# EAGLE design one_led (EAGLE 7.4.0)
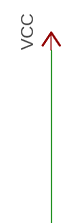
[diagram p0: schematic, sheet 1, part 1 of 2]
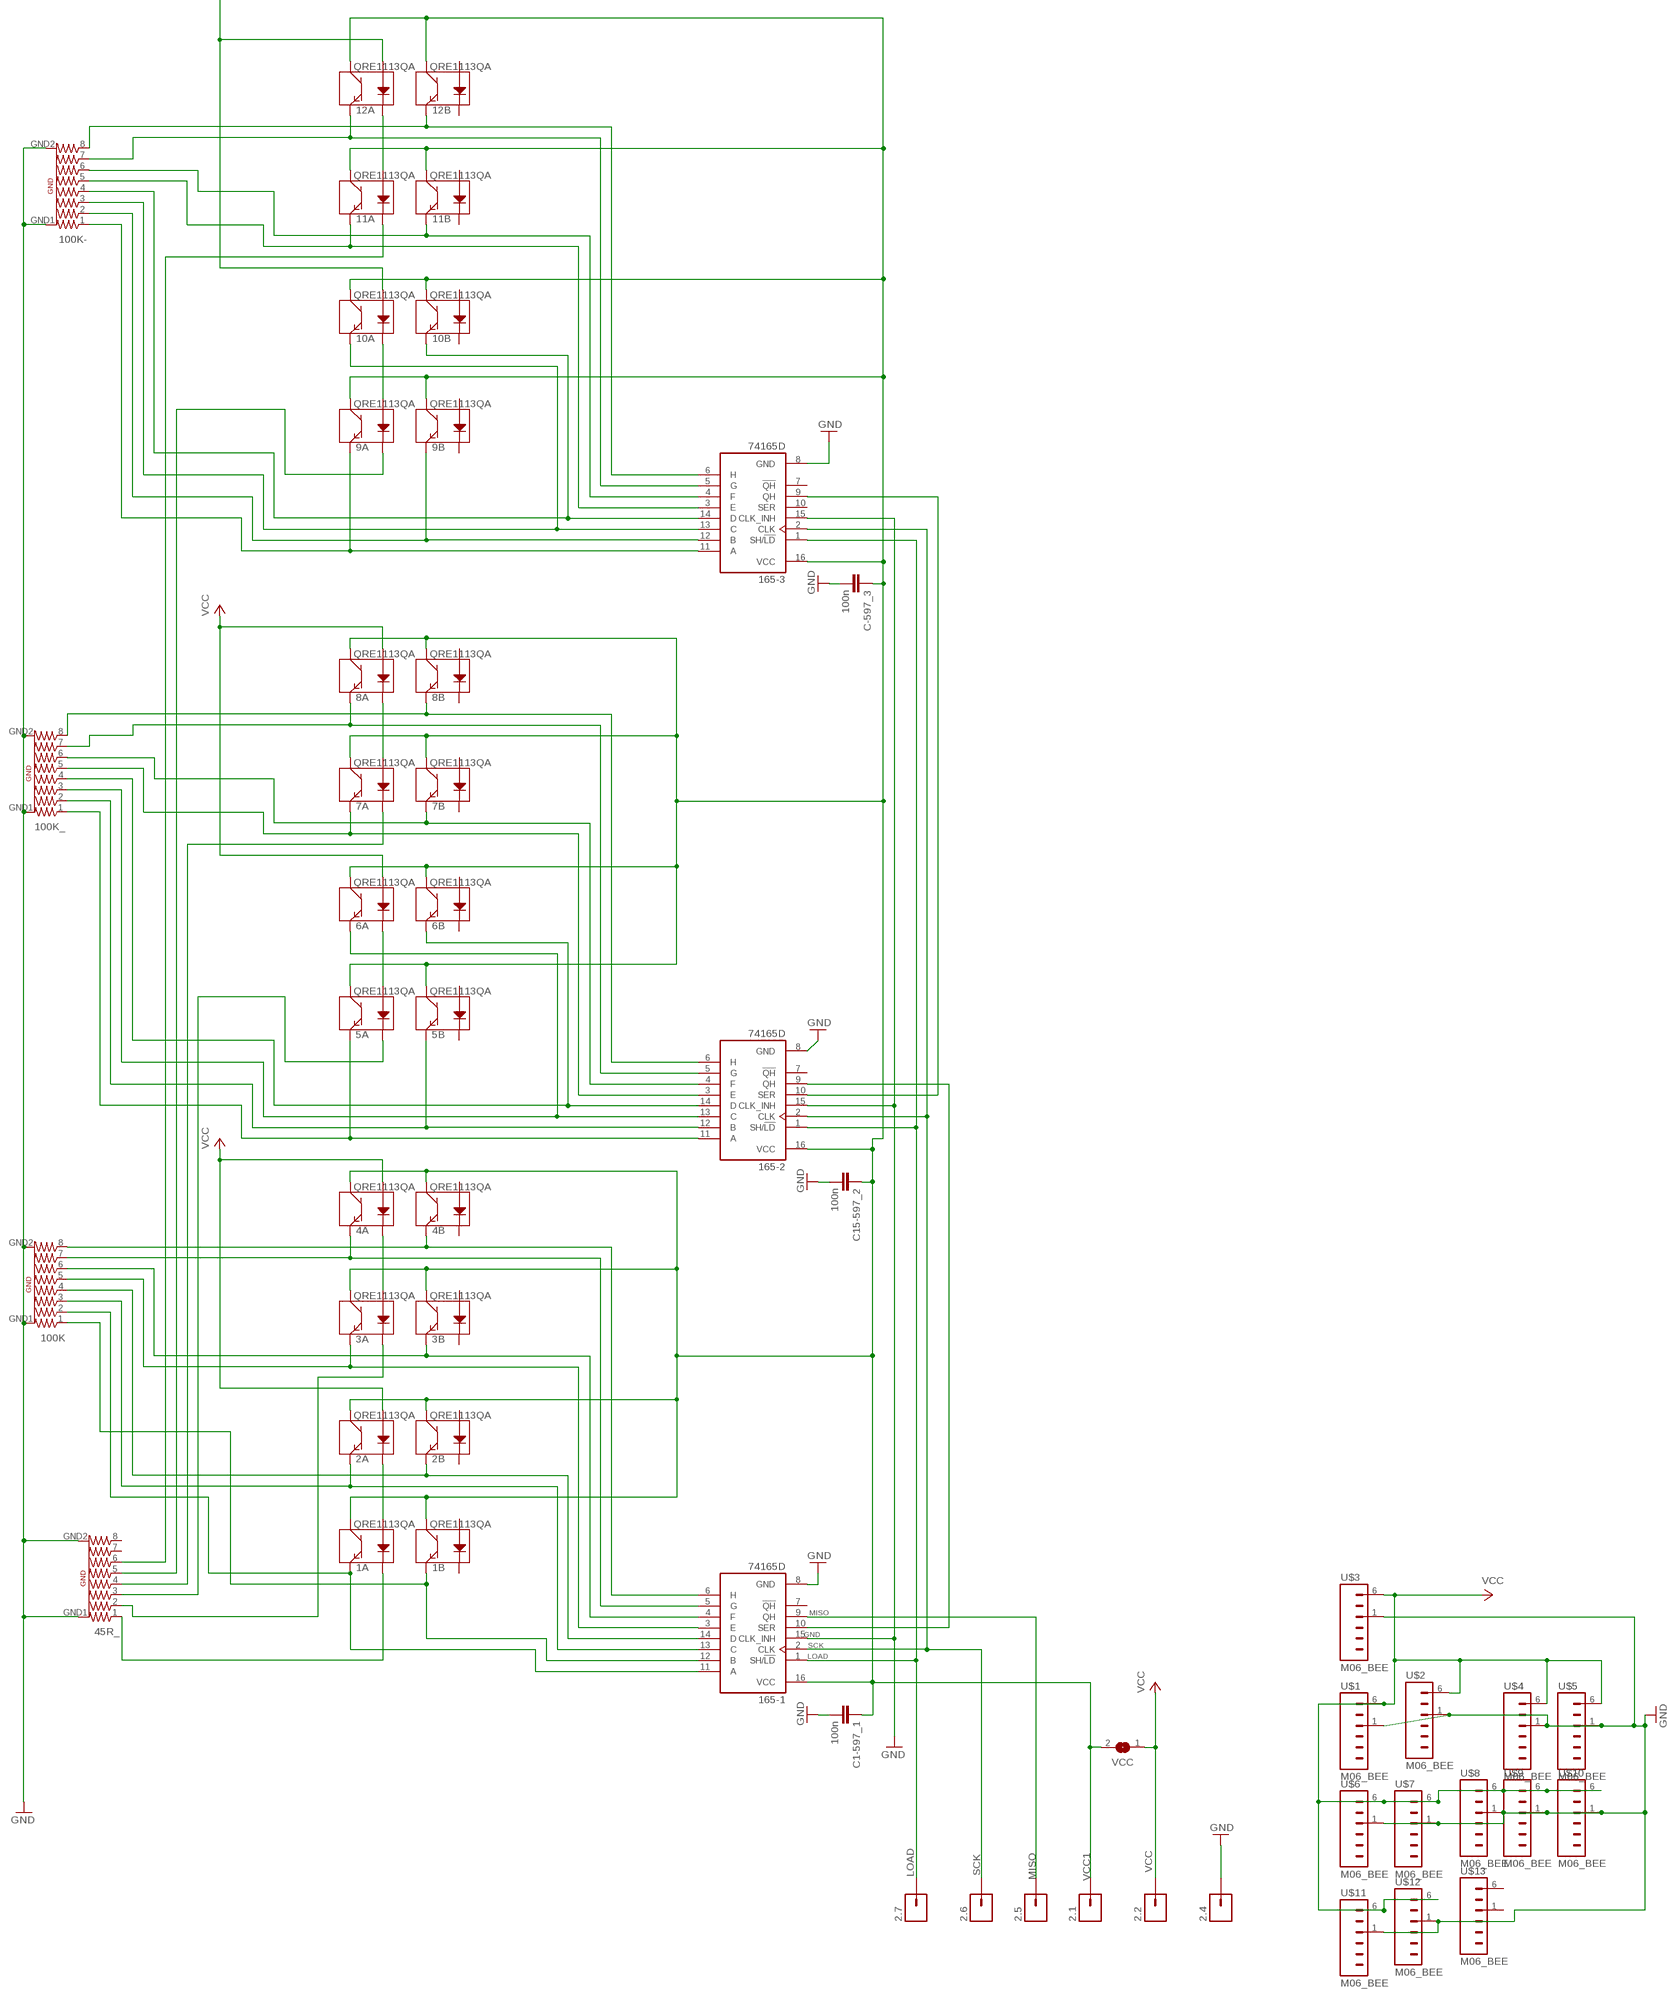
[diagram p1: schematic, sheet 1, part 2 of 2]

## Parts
1A  QRE1113QA  [QRE1113]
1B  QRE1113QA  [QRE1113]
2.1  M01ADN  [1X01-16GAUGE]
2.2  M01ADN  [1X01-16GAUGE]
2.4  M01ADN  [1X01-16GAUGE]
2.5  M01ADN  [1X01-16GAUGE]
2.6  M01ADN  [1X01-16GAUGE]
2.7  M01ADN  [1X01-16GAUGE]
2A  QRE1113QA  [QRE1113]
2B  QRE1113QA  [QRE1113]
3A  QRE1113QA  [QRE1113]
3B  QRE1113QA  [QRE1113]
4A  QRE1113QA  [QRE1113]
4B  QRE1113QA  [QRE1113]
5A  QRE1113QA  [QRE1113]
5B  QRE1113QA  [QRE1113]
6A  QRE1113QA  [QRE1113]
6B  QRE1113QA  [QRE1113]
7A  QRE1113QA  [QRE1113]
7B  QRE1113QA  [QRE1113]
8A  QRE1113QA  [QRE1113]
8B  QRE1113QA  [QRE1113]
9A  QRE1113QA  [QRE1113]
9B  QRE1113QA  [QRE1113]
10A  QRE1113QA  [QRE1113]
10B  QRE1113QA  [QRE1113]
11A  QRE1113QA  [QRE1113]
11B  QRE1113QA  [QRE1113]
12A  QRE1113QA  [QRE1113]
12B  QRE1113QA  [QRE1113]
45R_  RESISTOR-ARRAY_BUSSED  [1608_ARRAY]
100K  RESISTOR-ARRAY_BUSSED  [1608_ARRAY]
100K-  RESISTOR-ARRAY_BUSSED  [1608_ARRAY]
100K_  RESISTOR-ARRAY_BUSSED  [1608_ARRAY]
165-1  74165D  [SO16]
165-2  74165D  [SO16]
165-3  74165D  [SO16]
C1-597_1  100n  C-EUC0603  [C0603]
C15-597_2  100n  C-EUC0603  [C0603]
C-597_3  100n  C-EUC0603  [C0603]
U$1  M06_BEE  [1X06_BEE]
U$2  M06_BEE  [1X06_BEE]
U$3  M06_BEE  [1X06_BEE]
U$4  M06_BEE  [1X06_BEE]
U$5  M06_BEE  [1X06_BEE]
U$6  M06_BEE  [1X06_BEE]
U$7  M06_BEE  [1X06_BEE]
U$8  M06_BEE  [1X06_BEE]
U$9  M06_BEE  [1X06_BEE]
U$10  M06_BEE  [1X06_BEE]
U$11  M06_BEE  [1X06_BEE]
U$12  M06_BEE  [1X06_BEE]
U$13  M06_BEE  [1X06_BEE]
VCC  SJ  [SJ]

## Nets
GND: 2.4.1 45R_.GND1 45R_.GND2 100K-.GND1 100K-.GND2 100K.GND1 100K.GND2 100K_.GND1 100K_.GND2 165-1.8(GND) 165-1.15(CLK_INH) 165-2.8(GND) 165-2.15(CLK_INH) 165-3.8(GND) 165-3.15(CLK_INH) C1-597_1.2 C15-597_2.2 C-597_3.2 U$1.1 U$2.1 U$3.1 U$4.1 U$5.1 U$6.1 U$7.1 U$8.1 U$9.1 U$10.1 U$11.1 U$12.1
LOAD: 2.7.1 165-1.1(SH/!LD) 165-2.1(SH/!LD) 165-3.1(SH/!LD)
MISO: 2.5.1 165-1.9(QH)
N$18: 3A.4(E) 100K.5 165-1.3(E)
N$21: 165-2.10(SER) 165-3.9(QH)
N$30: 1A.4(E) 100K.2 165-1.11(A)
N$31: 3A.2(K) 45R_.2
N$34: 165-1.10(SER) 165-2.9(QH)
N$48: 1A.1(A) 2A.2(K)
N$56: 1A.2(K) 45R_.1
N$58: 3B.4(E) 100K.6 165-1.4(F)
N$74: 5A.1(A) 6A.2(K)
N$78: 6A.4(E) 100K_.3 165-2.13(C)
N$94: 5A.2(K) 45R_.3
N$100: 1B.4(E) 100K.1 165-1.12(B)
N$101: 2A.4(E) 100K.3 165-1.13(C)
N$102: 2B.4(E) 100K.4 165-1.14(D)
N$103: 3A.1(A) 4A.2(K)
N$105: 6B.4(E) 100K_.4 165-2.14(D)
N$107: 7A.1(A) 8A.2(K)
N$108: 4A.4(E) 100K.7 165-1.5(G)
N$109: 4B.4(E) 100K.8 165-1.6(H)
N$111: 8A.4(E) 100K_.7 165-2.5(G)
N$112: 8B.4(E) 100K_.8 165-2.6(H)
N$113: 7A.2(K) 45R_.4
N$115: 7A.4(E) 100K_.5 165-2.3(E)
N$117: 7B.4(E) 100K_.6 165-2.4(F)
N$118: 5B.4(E) 100K_.2 165-2.12(B)
N$119: 5A.4(E) 100K_.1 165-2.11(A)
N$127: 9A.1(A) 10A.2(K)
N$130: 10A.4(E) 100K-.3 165-3.13(C)
N$131: 10B.4(E) 100K-.4 165-3.14(D)
N$132: 11A.1(A) 12A.2(K)
N$134: 12A.4(E) 100K-.7 165-3.5(G)
N$135: 12B.4(E) 100K-.8 165-3.6(H)
N$136: 11A.2(K) 45R_.6
N$138: 11A.4(E) 100K-.5 165-3.3(E)
N$140: 11B.4(E) 100K-.6 165-3.4(F)
N$141: 9B.4(E) 100K-.2 165-3.12(B)
N$142: 9A.4(E) 100K-.1 165-3.11(A)
N$143: 9A.2(K) 45R_.5
SCK: 2.6.1 165-1.2(CLK) 165-2.2(CLK) 165-3.2(CLK)
VCC: 2.2.1 2A.1(A) 4A.1(A) 6A.1(A) 8A.1(A) 10A.1(A) 12A.1(A) U$1.6 U$2.6 U$3.6 U$4.6 U$5.6 U$6.6 U$7.6 U$8.6 U$9.6 U$10.6 U$11.6 U$12.6 VCC.1
VCC1: 1A.3(C) 1B.3(C) 2.1.1 2A.3(C) 2B.3(C) 3A.3(C) 3B.3(C) 4A.3(C) 4B.3(C) 5A.3(C) 5B.3(C) 6A.3(C) 6B.3(C) 7A.3(C) 7B.3(C) 8A.3(C) 8B.3(C) 9A.3(C) 9B.3(C) 10A.3(C) 10B.3(C) 11A.3(C) 11B.3(C) 12A.3(C) 12B.3(C) 165-1.16(VCC) 165-2.16(VCC) 165-3.16(VCC) C1-597_1.1 C15-597_2.1 C-597_3.1 VCC.2
Unconnected: 1B.1(A) 1B.2(K) 2B.1(A) 2B.2(K) 3B.1(A) 3B.2(K) 4B.1(A) 4B.2(K) 5B.1(A) 5B.2(K) 6B.1(A) 6B.2(K) 7B.1(A) 7B.2(K) 8B.1(A) 8B.2(K) 9B.1(A) 9B.2(K) 10B.1(A) 10B.2(K) 11B.1(A) 11B.2(K) 12B.1(A) 12B.2(K) 45R_.7 45R_.8 165-1.7(!QH) 165-2.7(!QH) 165-3.7(!QH) 165-3.10(SER) U$13.1 U$13.6

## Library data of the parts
1A 1B 2A 2B 3A 3B 4A 4B 5A 5B 6A 6B 7A 7B 8A 8B 9A 9B 10A 10B 11A 11B 12A 12B = BeeCounter2:QRE1113: Reflective object sensor
2.1 2.2 2.4-2.7 = OMSI - ADN:M01: Header 1
45R_ 100K 100K- 100K_ = Bee Counter 3:RESISTOR-ARRAY_BUSSED: Resistor Array <> http://industrial.panasonic.com/lecs/www-data/pdf/AOC0000/AOC0000CE3.pdf Digikey: U8470CT-ND Panasonic bussed EXB-E10
165-1-165-3 = SparkFun-DigitalIC:74*165
C1-597_1 C15-597_2 C-597_3 = resistor:C-EU: CAPACITOR, European symbol
U$1-U$13 = Bee Counter 3:M06_BEE
VCC = jumper:SJ: SMD solder JUMPER

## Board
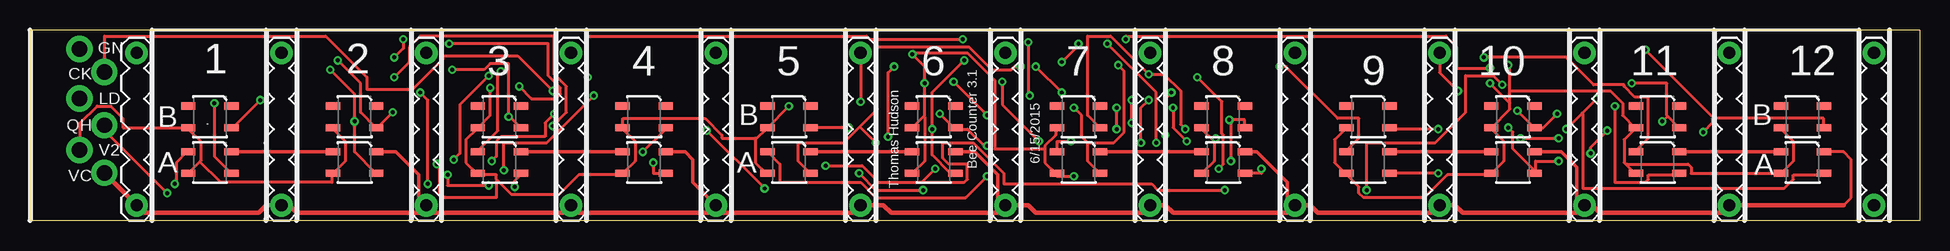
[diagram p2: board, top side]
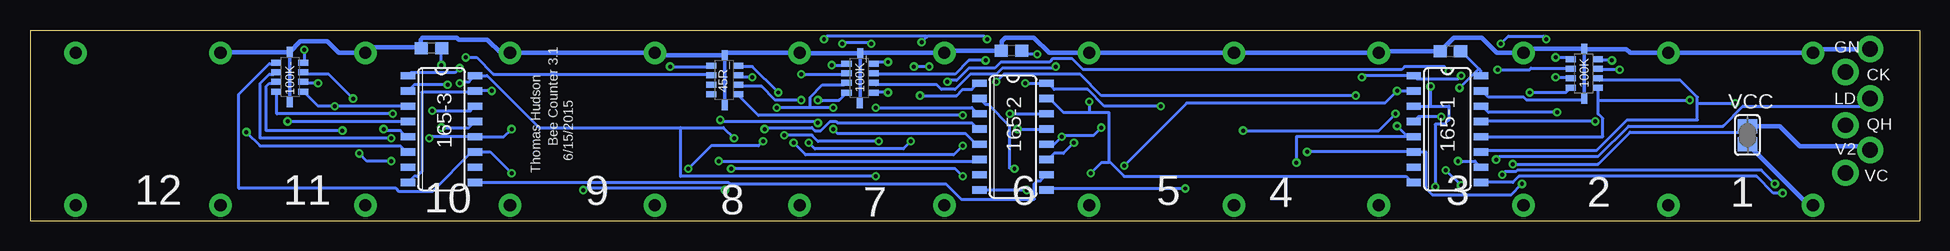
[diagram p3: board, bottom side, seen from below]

Size 157.48 x 15.88 mm. Coordinates in mm from the lower left corner, seen from the top.
Outline: 157.48,15.88 0,15.88 0,0 157.48,0 157.48,15.88
Copper layers (1*16): Top 0.0356mm / dielectric 1.5011mm / Bottom 0.0356mm
Design rules: minimum track width 10mil, minimum drill 13mil, track to track 6mil, track to pad 10mil, pad to pad 15mil, via to via 10mil, smd to smd 6mil, copper to edge 15mil, drill to drill 6mil, minimum pad ring 7mil, minimum via ring 7mil, stop-mask expansion 4mil, vias tented up to drill 25mil, thermal gap 10mil

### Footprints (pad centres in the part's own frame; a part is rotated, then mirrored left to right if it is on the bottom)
QRE1113 = smd 1.2 x 0.6: 1 -1.8,-0.9; 2 1.8,-0.9; 3 1.8,0.9; 4 -1.8,0.9
1X01-16GAUGE = drill 1.29 pad 2.184: 1 0,0
1608_ARRAY = smd 0.5 x 0.85: 1 -2.99,0.83; 2 -2.19,0.83; 3 -1.39,0.83; 4 -0.59,0.83; 5 -0.59,3.08; 6 -1.39,3.08; 7 -2.19,3.08; 8 -2.99,3.08 | smd 0.85 x 0.5: GND1 -3.88,1.96; GND2 0.28,1.94
SO16 = smd 0.6 x 1.2: 1 -4.445,-2.8; 2 -3.175,-2.8; 3 -1.905,-2.8; 4 -0.635,-2.8; 5 0.635,-2.8; 6 1.905,-2.8; 7 3.175,-2.8; 8 4.445,-2.8; 9 4.445,2.8; 10 3.175,2.8; 11 1.905,2.8; 12 0.635,2.8; 13 -0.635,2.8; 14 -1.905,2.8; 15 -3.175,2.8; 16 -4.445,2.8
C0603 = smd 1.1 x 1: 1 -0.85,0; 2 0.85,0
1X06_BEE = drill 1.016 pad 1.88: 1 -2.54,0; 6 10.16,0
SJ = smd 1.168 x 1.6: 1 -0.762,0; 2 0.762,0

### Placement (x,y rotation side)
1A  14.99,4.83 180 top
1B  14.99,8.64 180 top
2.1  4.13,5.87 0 top
2.2  6.19,3.97 0 top
2.4  4.13,14.29 0 top
2.5  6.19,7.94 0 top
2.6  6.19,12.38 0 top
2.7  4.13,10.16 0 top
2A  27.05,4.83 180 top
2B  27.05,8.64 180 top
3A  39.12,4.83 180 top
3B  39.12,8.64 180 top
4A  51.18,4.83 180 top
4B  51.18,8.64 180 top
5A  63.25,4.83 180 top
5B  63.25,8.64 180 top
6A  75.31,4.83 180 top
6B  75.31,8.64 180 top
7A  87.38,4.83 180 top
7B  87.38,8.64 180 top
8A  99.44,4.83 180 top
8B  99.44,8.64 180 top
9A  111.51,4.83 180 top
9B  111.51,8.64 180 top
10A  123.57,4.83 180 top
10B  123.57,8.64 180 top
11A  135.64,4.83 180 top
11B  135.64,8.64 180 top
12A  147.7,4.83 180 top
12B  147.7,8.64 180 top
45R_  97.63,13.49 90 bottom
100K  26,14.03 90 bottom
100K-  137.8,10.16 270 bottom
100K_  86.36,13.65 90 bottom
165-1  39.37,7.62 270 bottom
165-2  75.56,6.99 270 bottom
165-3  123.19,7.62 270 bottom
C1-597_1  75.69,14.16 180 bottom
C15-597_2  39.12,14.1 180 bottom
C-597_3  124.02,14.35 180 bottom
U$1  20.95,11.43 270 top
U$2  33.02,11.43 270 top
U$3  8.89,11.43 270 top
U$4  45.09,11.43 270 top
U$5  57.15,11.43 270 top
U$6  69.22,11.43 270 top
U$7  81.28,11.43 270 top
U$8  93.34,11.43 270 top
U$9  105.41,11.43 270 top
U$10  117.47,11.43 270 top
U$11  129.54,11.43 270 top
U$12  141.61,11.43 270 top
U$13  153.67,11.43 270 top
VCC  14.35,7.11 90 bottom

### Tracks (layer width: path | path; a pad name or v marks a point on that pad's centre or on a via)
GND  (via drill 0.33)
  Top 0.254: v74.42,2.54 70.49,2.54 v69.09,3.94 | v119,10.79 117.47,12.32 U$10.1 | U$6.1 v69.22,9.91
  Bottom 0.254: 165-1.8 42.29,3.17 42.8,3.68 66.29,3.68 67.5,4.89 | 67.5,4.89 67.56,4.95 67.56,9.02 69.22,9.02 | 69.22,9.02 71.37,9.02 72.52,10.16 165-2.15 | v74.42,2.54 165-2.8 | v69.09,3.94 68.2,4.83 67.56,4.83 67.5,4.89 | 165-3.8 125.48,3.68 125.22,3.68 124.84,4.06 124.84,10.67 120.52,10.67 165-3.15 v119,10.79 | 165-1.15 36.45,10.79 35.94,10.29 33.02,10.29 32.77,10.03 28.07,10.03 100K.GND1 | U$12.1 141.53,14.04 | v69.22,9.91 69.22,9.02
  Bottom 0.305: 27.92,14.29 100K.GND2 27.94,10.17 100K.GND1 | 76.52,14.19 C1-597_1.2 | 88.26,13.97 100K_.GND2 88.3,9.79 100K_.GND1 | 93.31,13.93 U$8.1 | 99.38,13.97 45R_.GND2 99.57,9.63 45R_.GND1 | 105.21,13.77 U$9.1 | U$10.1 118.27,13.97 | 124.94,14.42 C-597_3.2 | 100K-.GND1 135.84,9.9 100K-.GND2
  Bottom 0.381: 2.4.1 8.57,14.29 U$3.1 U$1.1 24.13,13.97 24.45,14.29 27.92,14.29 | 100K.GND2 32.68,14.31 U$2.1 35.24,13.97 36.51,15.24 38.82,15.24 C15-597_2.2 44.96,14.1 U$4.1 U$5.1 U$6.1 72.55,13.97 73.82,15.24 76.2,15.24 76.52,14.92 76.52,14.19 | C1-597_1.2 81.09,14.16 U$7.1 88.26,13.97 | 100K_.GND2 93.31,13.93 | U$8.1 99.38,13.97 | 45R_.GND2 105.21,13.77 | U$9.1 U$10.1 | 118.27,13.97 119.38,15.08 121.76,15.08 121.92,15.24 124.78,15.24 124.94,15.08 124.94,14.42 129.09,14.42 U$11.1 131.76,13.97 132.72,14.92 134.95,14.92 100K-.GND1 141.53,14.04
LOAD  (via drill 0.33)
  Top 0.254: v83.31,10.41 83.19,10.54 v83.19,14.86 | v77.72,15.11 69.98,15.11 69.72,15.37 46.48,15.37 v46.48,11.94 | v121.67,12.7 118.87,12.7 118.87,14.48 117.98,15.37 91.31,15.37 v91.31,15.11 | v35.31,5.08 35.81,5.59 35.81,9.65 v38.23,12.06
  Bottom 0.254: v83.31,10.41 80.26,10.41 79.76,10.92 78.99,10.92 78.49,11.43 165-2.1 | 82.74,15.3 82.68,15.37 77.98,15.37 v77.72,15.11 | 82.74,15.3 v83.19,14.86 | v46.48,11.94 46.35,12.06 165-1.1 41.91,11.81 38.48,11.81 v38.23,12.06 | v121.67,12.7 122.05,12.32 125.73,12.32 165-3.1 | v91.31,15.11 91.06,15.37 82.8,15.37 82.74,15.3 | v35.31,5.08 35.05,5.33 26.8,5.33 24.26,7.87 16.38,7.87 14.73,9.53 4.83,9.53 4.19,10.16 2.7.1
MISO  (via drill 0.33)
  Top 0.254: v11.43,2.29 6.22,7.49 6.22,7.87 2.5.1
  Bottom 0.254: 165-1.9 33.91,3.17 33.4,3.68 13.59,3.68 12.19,2.29 v11.43,2.29
N$18  (via drill 0.33)
  Top 0.254: v30.35,13.59 31.12,14.35 v31.12,15.11 | v34.92,14.73 43.18,14.73 43.18,12.06 44.2,11.05 44.2,10.54 43.81,10.16 41.78,10.16 v40.77,11.18 | v40.39,2.79 40.39,3.3 40.89,3.81 3A.4
  Bottom 0.254: v30.35,13.59 29.34,13.59 29.21,13.46 100K.5 | v31.12,15.11 31.37,15.37 34.29,15.37 v34.92,14.73 | 40.77,9.53 v40.77,11.18 | 165-1.3 40.77,9.53 | v40.39,2.79 40.39,8 39.62,8 39.24,8.38 39.24,9.53 40.77,9.53
N$21
  Bottom 0.254: 165-3.9 99.31,3.17 99.19,3.05 81.15,3.05 79.88,1.78 73.79,1.78 73.79,3.05 73.53,3.3 73.28,3.3 165-2.10
N$30  (via drill 0.33)
  Top 0.254: v15.37,9.78 15.37,5.33 16.76,3.94 1A.4
  Bottom 0.254: 18.54,9.78 18.54,8.38 24.38,8.38 26.92,5.84 36.32,5.84 36.45,5.71 165-1.11 | 18.54,9.78 18.54,10.29 19.94,11.68 26.67,11.68 26.8,11.81 100K.2 | 18.54,9.78 v15.37,9.78
N$31  (via drill 0.33)
  Top 0.254: v93.22,10.03 92.58,9.4 v92.58,6.48 | v84.07,6.6 81.03,9.65 v81.03,11.56 | v39.24,12.45 38.99,12.19 38.99,7.49 37.34,5.84 3A.2
  Bottom 0.254: v93.22,10.03 95.38,10.03 96.52,11.18 98.3,11.18 98.43,11.3 45R_.2 | v92.58,6.48 92.07,5.97 84.71,5.97 v84.07,6.6 | v81.03,11.56 80.9,11.68 80.26,11.68 79.25,12.7 77.09,12.7 76.58,13.21 72.52,13.21 72.26,13.46 70.61,13.46 69.72,12.57 43.18,12.57 42.93,12.83 39.62,12.83 v39.24,12.45
N$34  (via drill 0.33)
  Top 0.254: v38.48,4.95 38.86,5.33 38.86,6.6 39.24,6.99 42.93,6.99 42.93,8.13 v43.69,8.89 | v61.21,2.67 v56.39,7.49
  Bottom 0.254: v38.48,4.95 37.08,4.95 165-1.10 | v43.69,8.89 45.09,7.49 v56.39,7.49 | v61.21,2.67 72.52,2.67 72.64,2.54 165-2.9
N$48
  Top 0.305: 1A.1 2A.2
N$56  (via drill 0.33)
  Top 0.254: v76.96,11.56 v79.76,8.76 | v46.99,10.41 43.05,6.48 39.5,6.48 v39.5,4.19 | v38.23,2.92 34.8,2.92 v34.8,3.81 | v12.07,3.05 12.19,3.17 12.19,4.83 13.08,5.71 1A.2
  Bottom 0.254: v79.76,8.76 96.77,8.76 98.43,10.41 45R_.1 | v76.96,11.56 76.33,12.19 69.98,12.19 68.2,10.41 v46.99,10.41 | v38.23,2.92 v39.5,4.19 | v34.8,3.81 34.54,4.06 33.66,4.06 33.53,4.19 13.21,4.19 v12.07,3.05
N$58  (via drill 0.33)
  Top 0.254: v35.18,12.57 37.85,12.57 38.35,13.08 39.88,13.08 39.88,8.76 39.94,8.7 | 39.94,8.7 40.89,7.75 3B.4 | v39.88,8.64 39.94,8.7
  Bottom 0.254: v35.18,12.57 32.51,12.57 32.38,12.7 29.21,12.7 100K.6 | v39.88,8.64 41.78,8.64 165-1.4
N$74
  Top 0.305: 5A.1 6A.2
N$78  (via drill 0.33)
  Top 0.254: v77.85,13.34 75.18,10.67 v75.18,7.62 75.18,5.46 76.71,3.94 77.09,3.94 6A.4
  Bottom 0.254: v77.85,13.34 79.25,13.34 80.39,12.19 87.12,12.19 100K_.3 | v75.18,7.62 165-2.13
N$94  (via drill 0.33)
  Top 0.254: v97.28,11.94 99.31,9.91 99.31,7.24 99.44,7.11 99.44,4.7 v99.06,4.32 | v79.76,3.68 77.98,1.91 70.49,1.91 69.22,3.17 62.48,3.17 62.48,4.7 61.47,5.71 5A.2
  Bottom 0.254: v97.28,11.94 98.3,11.94 98.43,12.06 45R_.3 | v99.06,4.32 80.39,4.32 v79.76,3.68
N$100  (via drill 0.33)
  Top 0.254: v19.18,10.03 16.89,7.75 1B.4
  Bottom 0.254: 26.8,10.03 26.8,8.89 26.42,8.51 26.42,6.99 165-1.12 | 26.8,10.03 26.8,10.92 100K.1 | 26.8,10.03 v19.18,10.03
N$101  (via drill 0.33)
  Top 0.254: v25.02,12.57 27.05,10.54 v27.05,8.26 27.05,5.71 28.83,3.94 2A.4
  Bottom 0.254: v25.02,12.57 26.8,12.57 100K.3 | v27.05,8.26 165-1.13
N$102  (via drill 0.33)
  Top 0.254: v25.65,13.34 27.56,11.43 27.56,9.02 28.83,7.75 2B.4 28.96,7.75 v30.23,9.02
  Bottom 0.254: v25.65,13.34 26.8,13.34 100K.4 | v30.23,9.02 35.94,9.02 36.45,9.53 165-1.14
N$103
  Top 0.305: 3A.1 4A.2
N$105  (via drill 0.33)
  Top 0.254: v85.98,13.21 87.38,14.61 v87.38,14.73 | v89.79,14.73 93.85,10.67 v93.85,6.48 | v79.76,6.22 79.5,6.22 78.1,7.62 77.22,7.62 6B.4 77.09,7.62 v75.82,8.89
  Bottom 0.254: v85.98,13.21 87,13.21 87.12,13.08 100K_.4 | v87.38,14.73 87.5,14.86 89.66,14.86 v89.79,14.73 | v93.85,6.48 92.84,5.46 80.52,5.46 v79.76,6.22 | v75.82,8.89 165-2.14
N$107
  Top 0.305: 7A.1 8A.2
N$108  (via drill 0.33)
  Top 0.254: v30.35,11.94 31.62,13.21 31.62,14.48 32.51,15.37 43.69,15.37 43.69,12.19 44.7,11.18 44.7,9.02 v43.56,7.87 | v51.94,4.83 51.94,3.94 52.96,3.94 4A.4
  Bottom 0.254: v30.35,11.94 29.21,11.94 100K.7 | 42.74,7.05 42.67,6.99 165-1.5 | 42.74,7.05 v43.56,7.87 | v51.94,4.83 51.94,6.99 42.8,6.99 42.74,7.05
N$109  (via drill 0.33)
  Top 0.254: v32.51,10.67 33.15,10.03 v33.15,3.05 | v51.05,5.71 52.96,7.62 4B.4
  Bottom 0.254: v32.51,10.67 29.46,10.67 29.21,10.92 100K.8 | v33.15,3.05 34.04,2.16 40.64,2.16 41.15,2.67 41.15,5.71 165-1.6 v51.05,5.71
N$111  (via drill 0.33)
  Top 0.254: v90.55,7.62 v90.55,9.4 | v102.62,4.32 102.62,3.94 101.35,3.94 8A.4 | v96.39,6.6 95.25,7.75 v95.25,9.4
  Bottom 0.254: 92.46,9.4 92.46,10.29 91.44,11.3 89.66,11.3 89.53,11.43 100K_.7 | v90.55,9.4 92.46,9.4 | v90.55,7.62 90.17,7.24 79.5,7.24 78.61,6.35 165-2.5 | v102.62,4.32 100.71,6.22 96.77,6.22 v96.39,6.6 | 92.46,9.4 v95.25,9.4
N$112  (via drill 0.33)
  Top 0.254: v91.82,8.13 v91.82,10.03 | 100.08,8.38 101.22,8.38 101.22,7.75 8B.4 | 100.08,8.38 v100.08,4.95 | 100.08,8.38 v99.95,8.38
  Bottom 0.254: v91.82,10.03 90.04,10.03 89.53,10.54 100K_.8 | v91.82,8.13 91.95,8.26 99.82,8.26 v99.95,8.38 | v100.08,4.95 78.61,4.95 78.49,5.08 165-2.6
N$113  (via drill 0.33)
  Top 0.254: v95.12,10.67 94.62,10.16 v94.62,7.11 | v86.74,6.6 85.6,6.6 85.6,5.84 7A.2
  Bottom 0.254: v95.12,10.67 97.28,12.83 98.43,12.83 45R_.4 | v94.62,7.11 92.33,7.11 91.82,6.6 v86.74,6.6
N$115  (via drill 0.33)
  Top 0.254: v90.68,12.95 91.19,12.45 91.19,7.37 90.3,6.48 88.14,6.48 | 88.14,6.48 88.14,4.95 89.15,3.94 7A.4 | v87,9.4 87.63,8.76 87.63,6.99 88.14,6.48
  Bottom 0.254: v90.68,12.95 89.53,12.95 100K_.5 | v87,9.4 78.99,9.4 78.49,8.89 165-2.3
N$117  (via drill 0.33)
  Top 0.254: 7B.4 89.15,7.75 88.14,8.76 88.14,15.37 90.04,15.37 v93.22,12.19 94.49,12.19 95.88,10.79 95.88,8 v96.27,7.62
  Bottom 0.254: v93.22,12.19 89.53,12.19 100K_.6 | v96.27,7.62 96.14,7.75 92.33,7.75 92.07,7.49 91.57,7.49 90.81,8.26 90.3,8.26 90.17,8.13 78.99,8.13 78.49,7.62 165-2.4
N$118  (via drill 0.33)
  Top 0.254: v72.01,12.83 71.5,12.32 v71.5,6.99 | v68.2,7.75 65.15,7.75 5B.4
  Bottom 0.254: v72.01,12.83 72.14,12.7 76.45,12.7 76.96,12.19 79.12,12.19 80.39,10.92 81.53,10.92 81.91,11.3 87,11.3 87.12,11.43 100K_.2 | 165-2.12 72.14,6.35 v71.5,6.99 71.37,7.11 68.83,7.11 v68.2,7.75
N$119  (via drill 0.33)
  Top 0.254: v83.82,12.83 v85.98,10.67 | v82.55,12.83 82.04,12.83 81.79,12.57 80.14,12.57 78.23,14.48 70.61,14.48 70.61,9.27 69.15,7.81 | 69.15,7.81 67.82,6.48 64.01,6.48 64.01,4.95 65.02,3.94 5A.4 | 69.15,7.81 v70.49,6.48
  Bottom 0.254: v85.98,10.67 87.12,10.67 100K_.1 | v82.55,12.83 v83.82,12.83 | v70.49,6.48 71.37,5.59 72.14,5.59 72.64,5.08 165-2.11
N$127
  Top 0.305: 9A.1 10A.2
N$130  (via drill 0.33)
  Top 0.254: v131.44,7.49 130.05,6.1 v130.05,5.59 | v127.38,4.95 125.48,4.95 125.48,4.06 | 125.48,4.06 125.48,3.94 10A.4 125.48,4.06 | v123.19,7.75 123.57,7.37 123.57,5.97 125.48,4.06
  Bottom 0.254: v131.44,7.49 137.8,7.49 137.8,11.18 137.54,11.43 137.03,11.43 100K-.3 | v130.05,5.59 129.41,4.95 v127.38,4.95 | v123.19,7.75 120.9,7.75 165-3.13
N$131  (via drill 0.33)
  Top 0.254: v127.25,8.89 126.11,7.75 125.48,7.75 10B.4 125.35,7.75 v123.95,9.14
  Bottom 0.254: v127.25,8.89 136.91,8.89 136.91,10.67 100K-.4 | v123.95,9.14 120.78,9.14 165-3.14
N$132
  Top 0.305: 11A.1 12A.2
N$134  (via drill 0.33)
  Top 0.254: v128.02,7.62 129.35,8.95 | 129.35,8.95 v130.56,10.16 | 12A.4 149.48,3.81 146.94,3.81 146.94,3.43 146.18,2.67 129.41,2.67 129.41,8.89 129.35,8.95
  Bottom 0.254: v130.56,10.16 132.59,12.19 134.49,12.19 134.62,12.32 100K-.7 | v128.02,7.62 127.89,7.49 126.62,7.49 126.11,6.99 165-3.5
N$135  (via drill 0.33)
  Top 0.254: 140.27,8.57 140.34,8.51 149.48,8.51 149.48,7.75 12B.4 | 140.27,8.57 v134.62,14.22 | v139.45,7.37 140.21,8.13 140.21,8.51 140.27,8.57
  Bottom 0.254: v134.62,14.22 134.62,13.21 100K-.8 | v139.45,7.37 138.3,6.22 126.62,6.22 126.11,5.71 165-3.6
N$136  (via drill 0.33)
  Top 0.254: v121.16,13.59 128.14,13.59 128.14,13.46 130.3,11.3 132.84,11.3 132.84,11.18 133.73,10.29 134.87,10.29 134.87,6.86 133.86,5.84 11A.2
  Bottom 0.254: v121.16,13.59 120.27,13.59 118.87,12.19 100.84,12.19 45R_.6
N$138  (via drill 0.33)
  Top 0.254: v132.08,9.53 132.08,3.17 134.62,3.17 134.87,3.43 134.87,3.81 137.41,3.81 11A.4
  Bottom 0.254: 165-3.3 v132.08,9.53 133.48,9.53 134.62,10.67 100K-.5
N$140  (via drill 0.33)
  Top 0.254: v133.48,11.43 136.4,11.43 136.4,8.76 136.46,8.7 | 136.46,8.7 137.41,7.75 11B.4 | 136.46,8.7 v136.02,8.26
  Bottom 0.254: v133.48,11.43 134.62,11.43 100K-.6 | v136.02,8.26 165-3.4
N$141  (via drill 0.33)
  Top 0.254: v124.21,6.86 v127.38,6.86 | v117.35,7.62 113.41,7.62 9B.4
  Bottom 0.254: v127.38,6.86 138.3,6.86 138.3,11.43 137.54,12.19 137.16,12.19 137.03,12.32 100K-.2 | v124.21,6.86 124.08,6.99 165-3.12 117.98,6.99 v117.35,7.62
N$142  (via drill 0.33)
  Top 0.254: v117.35,3.94 113.41,3.94 9A.4
  Bottom 0.254: 100K-.1 137.03,13.08 137.54,13.08 140.08,10.54 140.08,2.67 127,2.67 126.75,2.41 123.95,2.41 120.65,5.71 165-3.11 119.13,5.71 v117.35,3.94
N$143  (via drill 0.33)
  Top 0.254: v104.14,12.83 104.65,12.83 108.97,8.51 110.74,8.51 110.74,6.86 109.73,5.84 9A.2
  Bottom 0.254: v104.14,12.83 100.84,12.83 45R_.5
SCK  (via drill 0.33)
  Top 0.254: v43.56,10.79 40.64,13.72 34.42,13.72 34.42,13.46 31.88,10.92 28.07,10.92 28.07,11.94 24.64,15.37 6.22,15.37 6.22,12.45 2.6.1 | 74.36,3.24 74.29,3.17 70.49,3.17 70.49,3.43 69.34,4.57 v66.29,4.57 | 74.36,3.24 v75.44,4.32 | v122.68,11.3 121.92,12.06 119.63,12.06 119.63,9.02 117.09,6.48 111.38,6.48 v111.38,2.54 | v99.57,2.54 93.98,2.54 93.47,3.05 81.15,3.05 81.15,3.94 78.61,6.48 76.07,6.48 76.07,5.21 76.58,4.7 78.1,4.7 78.1,3.43 77.85,3.17 74.42,3.17 74.36,3.24
  Bottom 0.254: 165-1.2 v43.56,10.79 44.58,9.78 61.09,9.78 v66.29,4.57 | v75.44,4.32 75.82,4.32 75.82,7.87 77.6,9.65 77.85,9.65 165-2.2 | v122.68,11.3 125.48,11.3 165-3.2 | v111.38,2.54 111.25,2.67 99.69,2.67 v99.57,2.54
VCC
  Top 0.254: 151.13,1.27 151.77,1.91 151.77,5.08 151.13,5.71 149.51,5.71 12A.1
  Top 0.305: 2A.1 30.47,5.73 32.38,3.81 32.38,1.91 U$2.6 | 4A.1 54.6,5.73 55.24,5.08 55.24,3.17 U$5.6 | 6A.1 78.73,5.73 80.65,3.81 80.65,1.91 U$7.6 | 8A.1 102.22,5.73 104.78,3.17 104.78,1.91 U$9.6 | 10A.1 127.62,5.73 128.91,4.45 128.91,1.91 U$11.6
  Top 0.381: 151.13,1.27 U$12.6 140.97,0.64 130.81,0.64 130.18,1.27 U$11.6 128.91,0.64 119.38,0.64 118.75,1.27 U$10.6 116.84,0.64 107.31,0.64 106.68,1.27 U$9.6 104.78,0.64 95.25,0.64 94.62,1.27 U$8.6 92.71,0.64 83.82,0.64 83.19,1.27 U$7.6 80.65,0.64 71.75,0.64 71.12,1.27 U$6.6 68.58,0.64 57.78,0.64 U$5.6 56.52,0.64 45.72,0.64 U$4.6 44.45,0.64 33.66,0.64 U$2.6 32.38,0.64 22.23,0.64 21.59,1.27 U$1.6 19.68,1.27 19.05,0.64 9.53,0.64 U$3.6 2.2.1
  Bottom 0.381: U$3.6 9.27,1.27 VCC.1
VCC1  (via drill 0.33)
  Top 0.254: 12B.3 145.92,7.62 146.94,6.6 146.94,4.95 145.92,3.94 12A.3 145.8,3.94 138.43,3.94 138.43,4.45 138.18,4.7 133.1,4.7 133.03,4.64 | 98.62,6.67 97.66,7.62 8B.3 | 98.62,6.67 98.68,6.6 98.68,4.95 97.66,3.94 8A.3 | 133.03,4.64 132.84,4.83 132.84,6.73 133.73,7.62 11B.3 133.73,7.75 132.72,8.76 132.72,9.78 131.7,10.79 123.32,10.79 | 133.03,4.64 133.73,3.94 11A.3 | 9B.3 109.6,7.62 108.71,6.73 108.71,4.83 109.6,3.94 9A.3 109.73,3.81 110.74,2.79 110.74,2.29 111.12,1.91 116.21,1.91 118.11,3.81 121.67,3.81 10A.3 121.79,3.94 122.81,4.95 122.81,6.6 121.79,7.62 10B.3 121.79,7.75 123.32,9.27 123.32,9.78 | v123.19,12.95 123.32,12.83 123.32,10.79 | 123.32,9.78 123.32,10.79 | 123.32,9.78 v121.67,11.43 | v98.81,6.86 98.62,6.67 | 14.16,4.89 14.22,4.95 14.22,6.6 13.21,7.62 1B.3 13.08,7.75 7.75,7.75 7.75,8.51 6.73,9.53 5.59,9.53 4.19,8.13 4.19,5.97 2.1.1 | 14.16,4.89 13.21,3.94 1A.3 | 2B.3 25.27,7.62 26.29,6.6 26.29,4.95 25.27,3.94 2A.3 25.15,3.81 25.15,3.17 15.88,3.17 14.16,4.89 | 84.58,5.97 84.58,6.22 85.47,7.11 85.47,7.62 7B.3 | 84.58,5.97 84.58,4.83 85.47,3.94 7A.3 85.6,3.81 85.6,3.68 v87,3.68 | 74.49,8.7 73.53,7.75 6B.3 | 74.49,8.7 74.55,8.76 v74.55,11.43 74.55,12.83 v73.53,13.84 73.66,13.84 73.66,13.97 78.1,13.97 80.39,11.68 80.39,5.97 84.58,5.97 | 6A.3 73.53,3.94 74.55,4.95 74.55,8.64 74.49,8.7 | v38.35,11.05 38.35,8.76 37.34,7.75 3B.3 37.21,7.62 36.32,6.73 36.32,4.83 37.21,3.94 3A.3 37.34,3.81 38.86,3.81 38.86,3.43 38.92,3.37 | 60.51,6.79 61.34,7.62 5B.3 61.47,7.75 v63.25,9.53 | 60.51,6.79 60.45,6.73 60.45,4.83 61.34,3.94 5A.3 | 60.51,6.79 60.45,6.86 57.66,6.86 57.66,7.11 56.26,8.51 49.4,8.51 49.4,7.75 4B.3 49.4,7.62 50.42,6.6 50.42,4.95 49.4,3.94 4A.3 49.28,3.81 45.72,3.81 44.07,2.16 40.13,2.16 38.92,3.37
  Top 0.254: v33.91,4.7 34.16,4.45 34.16,2.29 34.54,1.91 38.86,1.91 38.86,3.3 38.92,3.37
  Bottom 0.254: v123.19,12.95 123.19,14.35 C-597_3.1 | v121.67,11.43 121.54,11.56 120.9,11.56 165-3.16 119.38,12.06 115.06,7.75 103.25,7.75 | v98.81,6.86 99.69,7.75 103.25,7.75 | v73.53,13.84 74.55,13.84 74.8,14.1 C1-597_1.1 | v74.55,11.43 165-2.16 72.64,11.43 72.14,10.92 69.34,10.92 67.94,9.53 v63.25,9.53 | 36.77,12.64 36.58,12.45 165-1.16 | 36.77,12.64 38.23,14.1 C15-597_2.1 | v38.35,11.05 36.77,12.64 | VCC.2 14.86,7.37 24.13,7.37 26.8,4.7 v33.91,4.7 | 103.25,7.75 103.25,3.68 v87,3.68
  Bottom 0.381: VCC.2 11.68,7.87 10,6.19 4.45,6.19 2.1.1

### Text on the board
tPlace: Bee Counter 3.1 | 1 | 2 | 3 | 4 | 5 | 6 | 7 | 8 | 10 | 11 | 12 | 9 | 6/15/2015 | B | B | B | A | A | A | Thomas Hudson
bPlace: Bee Counter 3.1 | 6/15/2015 | 1 | 2 | 3 | 4 | 5 | 6 | 9 | Thomas Hudson | 11 | 12 | 7 | 8 | 10
tNames: GN | CK | LD | QH | V2 | VC
bNames: GN | CK | LD | QH | V2 | VC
